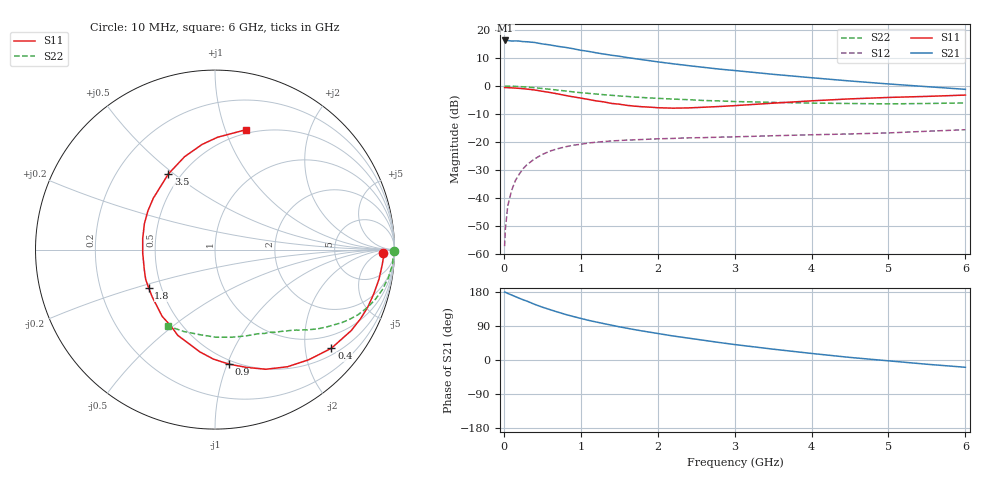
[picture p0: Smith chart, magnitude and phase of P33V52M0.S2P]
! SIEMENS Small Signal Semiconductors
! BFP181
! Si NPN RF Bipolar Junction Transistor in SOT143
! VCE = 3.5 V  IC = 2 mA
! Common Emitter S-Parameters:  March  1996
# GHz  S  MA  R  50
!  f  S11  S21  S12  S22
! GHz  MAG  ANG  MAG  ANG  MAG  ANG  MAG  ANG
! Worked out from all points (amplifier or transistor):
!   36 points, 10 MHz to 6 GHz, reference 50 ohm
!   highest |S21| = 16.2 dB at 20 MHz (marker M1)
!   |S21| within 3 dB of that: start of sweep to 910.9 MHz
!   unconditionally stable (mu >= 1): 2.482 GHz to end of sweep
!   at 250 MHz: K = 0.13, MSG = 22.7 dB, |S12| = -29.5 dB
!   at 1.4 GHz: K = 0.64, MSG = 15.3 dB, |S12| = -19.6 dB
!   at 6 GHz: K = 1.15, MAG = 4.9 dB, |S12| = -15.6 dB
!   lowest NFmin = 1.35 dB at 450 MHz
!   S11 on the Smith chart (normalised r, x): 10 MHz: 27, -9; 400 MHz: 0.65, -2.58; 900 MHz: 0.47, -1.01; 1.8 GHz: 0.43, -0.22; 3.5 GHz: 0.43, +0.48; 6 GHz: 0.46, +1.18
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0.01  0.9363 -1.3  6.412 179.2  0.0014 86.1  0.9975 -0.4
0.02  0.9403 -2.1  6.49 178.8  0.0028 86.9  0.9908 -0.9
0.05  0.9358 -5.1  6.479 175.7  0.0072 89.7  0.9933 -2.3
0.1  0.9283 -10.3  6.336 171.6  0.0137 82.3  0.9929 -4.7
0.15  0.9182 -15.6  6.371 167.3  0.0206 80.3  0.9852 -6.9
0.25  0.8978 -25.4  6.188 158.9  0.0336 74.8  0.9677 -11.4
0.3  0.8831 -30.7  6.151 155.4  0.0396 71.9  0.9587 -13.5
0.4  0.85 -40.3  5.974 146.9  0.0504 65.9  0.9334 -17.6
0.5  0.8058 -49.6  5.633 139.5  0.0603 60.5  0.9037 -21.3
0.6  0.7673 -58.3  5.403 132.9  0.0693 56.2  0.8754 -24.5
0.8  0.6792 -75.1  4.889 120.4  0.0826 48.0  0.8158 -29.9
0.9  0.6425 -83.1  4.627 114.9  0.0881 44.7  0.7868 -32.1
1.1  0.5762 -98.4  4.148 104.7  0.0964 38.9  0.7398 -36.1
1.3  0.5212 -113.4  3.714 96.0  0.1024 34.5  0.7003 -39.4
1.5  0.4749 -128.2  3.393 87.6  0.1068 31.0  0.6654 -42.2
1.8  0.4272 -149.9  2.947 76.6  0.1115 27.1  0.6242 -46.0
2.2  0.4033 -177.2  2.492 63.4  0.1165 23.1  0.5851 -51.2
2.8  0.4316 150.0  2.003 46.2  0.1227 19.2  0.5431 -59.3
3.5  0.495 121.7  1.618 28.6  0.13 16.5  0.5113 -70.0
4.5  0.5904 97.0  1.23 6.8  0.14 13.0  0.4881 -89.6
5.5  0.6535 81.8  0.975 -11.2  0.1563 11.6  0.4882 -110.8
6  0.69 75.5  0.873 -19.2  0.1665 9.7  0.5003 -121.8
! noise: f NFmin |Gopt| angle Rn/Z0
0.45  1.35  0.6  17  0.4
0.9  1.45  0.5  36  0.4
1.8  1.8  0.31  80  0.37
